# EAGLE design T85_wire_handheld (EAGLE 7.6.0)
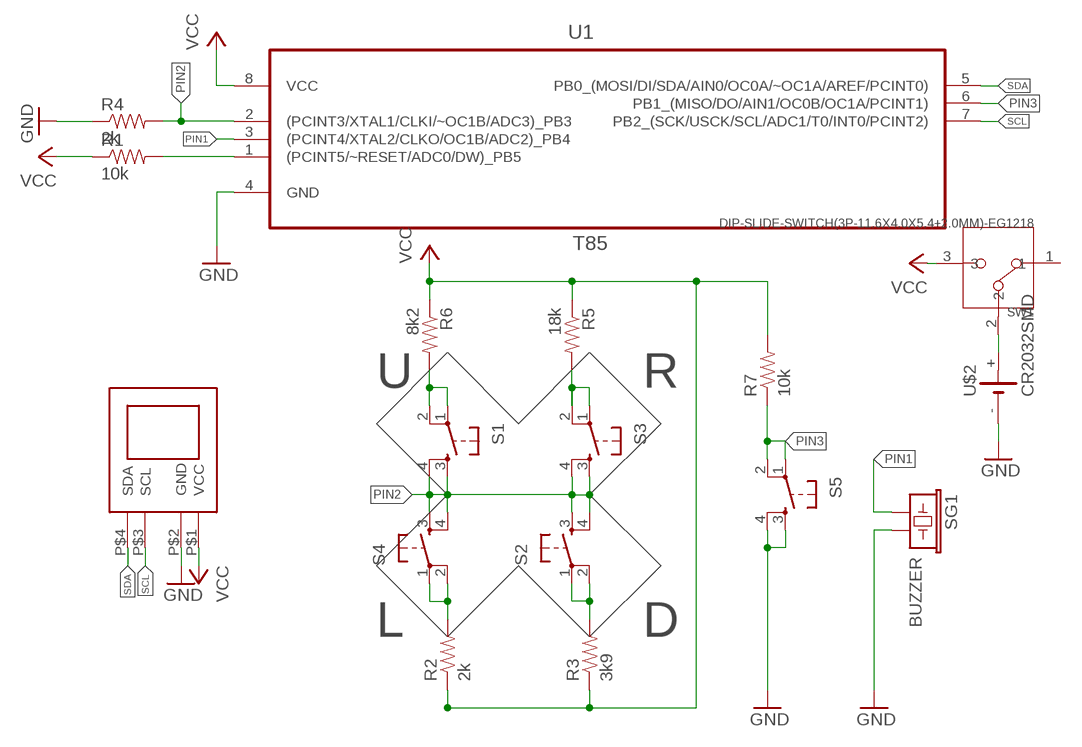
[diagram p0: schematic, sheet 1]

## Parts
R1  10k  RESISTOREZ  [AXIAL-0.3EZ]
R2  2k  RESISTOREZ  [AXIAL-0.3EZ]
R3  3k9  RESISTOREZ  [AXIAL-0.3EZ]
R4  2k  RESISTOREZ  [AXIAL-0.3EZ]
R5  18k  RESISTOREZ  [AXIAL-0.3EZ]
R6  8k2  RESISTOREZ  [AXIAL-0.3EZ]
R7  10k  RESISTOREZ  [AXIAL-0.3EZ]
S1  TAC_SWITCHPTH  [TACTILE-PTH]
S2  TAC_SWITCHPTH  [TACTILE-PTH]
S3  TAC_SWITCHPTH  [TACTILE-PTH]
S4  TAC_SWITCHPTH  [TACTILE-PTH]
S5  TAC_SWITCHPTH  [TACTILE-PTH]
SG1  BUZZER  BUZZERNS  [BUZZER-12MM-NS]
SW1  DIP-SLIDE-SWITCH(3P-11.6X4.0X5.4+2.0MM)-EG1218  [SW3-2.5-11.6X4.0X5.4+2.0MM]
U1  T85  MCU-ATTINY85-20PU(DIP8)1  [DIP254P762X533-8]
U$1  OLED_I2C_VGCD  [OLED_1.3]
U$2  CR2032SMD  [CR2032SMD]

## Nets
GND: R4.P$1 S5.3 S5.4 SG1.- U1.4(GND) U$1.P$2(GND) U$2.-
N$1: R6.P$2 S1.1 S1.2
N$2: R5.P$2 S3.1 S3.2
N$3: SW1.2 U$2.+
N$10: R3.P$2 S2.1 S2.2
N$11: R1.P$2 U1.1((PCINT5/~RESET/ADC0/DW)_PB5)
N$12: R2.P$2 S4.1 S4.2
PIN1: SG1.+ U1.3((PCINT4/XTAL2/CLKO/OC1B/ADC2)_PB4)
PIN2: R4.P$2 S1.3 S1.4 S2.3 S2.4 S3.3 S3.4 S4.3 S4.4 U1.2((PCINT3/XTAL1/CLKI/~OC1B/ADC3)_PB3)
PIN3: R7.P$1 S5.1 S5.2 U1.6(PB1_(MISO/DO/AIN1/OC0B/OC1A/PCINT1))
SCL: U1.7(PB2_(SCK/USCK/SCL/ADC1/T0/INT0/PCINT2)) U$1.P$3(SCL)
SDA: U1.5(PB0_(MOSI/DI/SDA/AIN0/OC0A/~OC1A/AREF/PCINT0)) U$1.P$4(SDA)
VCC: R1.P$1 R2.P$1 R3.P$1 R5.P$1 R6.P$1 R7.P$2 SW1.3 U1.8(VCC) U$1.P$1(VCC)
Unconnected: SW1.1

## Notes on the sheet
- U | R
- L | D

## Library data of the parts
R1-R7 = SparkFun-Passives:RESISTOR: Resistor
S1-S5 = SparkFun-Electromechanical:TAC_SWITCH: Momentary Switch Button commonly used for reset or general input. Spark Fun Electronics SKU : COM-00097 SMT- SWCH-08247
SG1 = SparkFun-Electromechanical:BUZZER: Buzzer 12mm
SW1 = Seeed-OPL-Switch:DIP-SLIDE-SWITCH(3P-11.6X4.0X5.4+2.0MM): 311010006
U1 = Seeed-OPL-ic:MCU-ATTINY85-20PU(DIP8): 310010112; MPN: ATTINY85-20PU; VALUE: ATTINY85-20PU-DIP8
U$1 = oled:OLED_I2C_VGCD
U$2 = battery:CR2032SMD

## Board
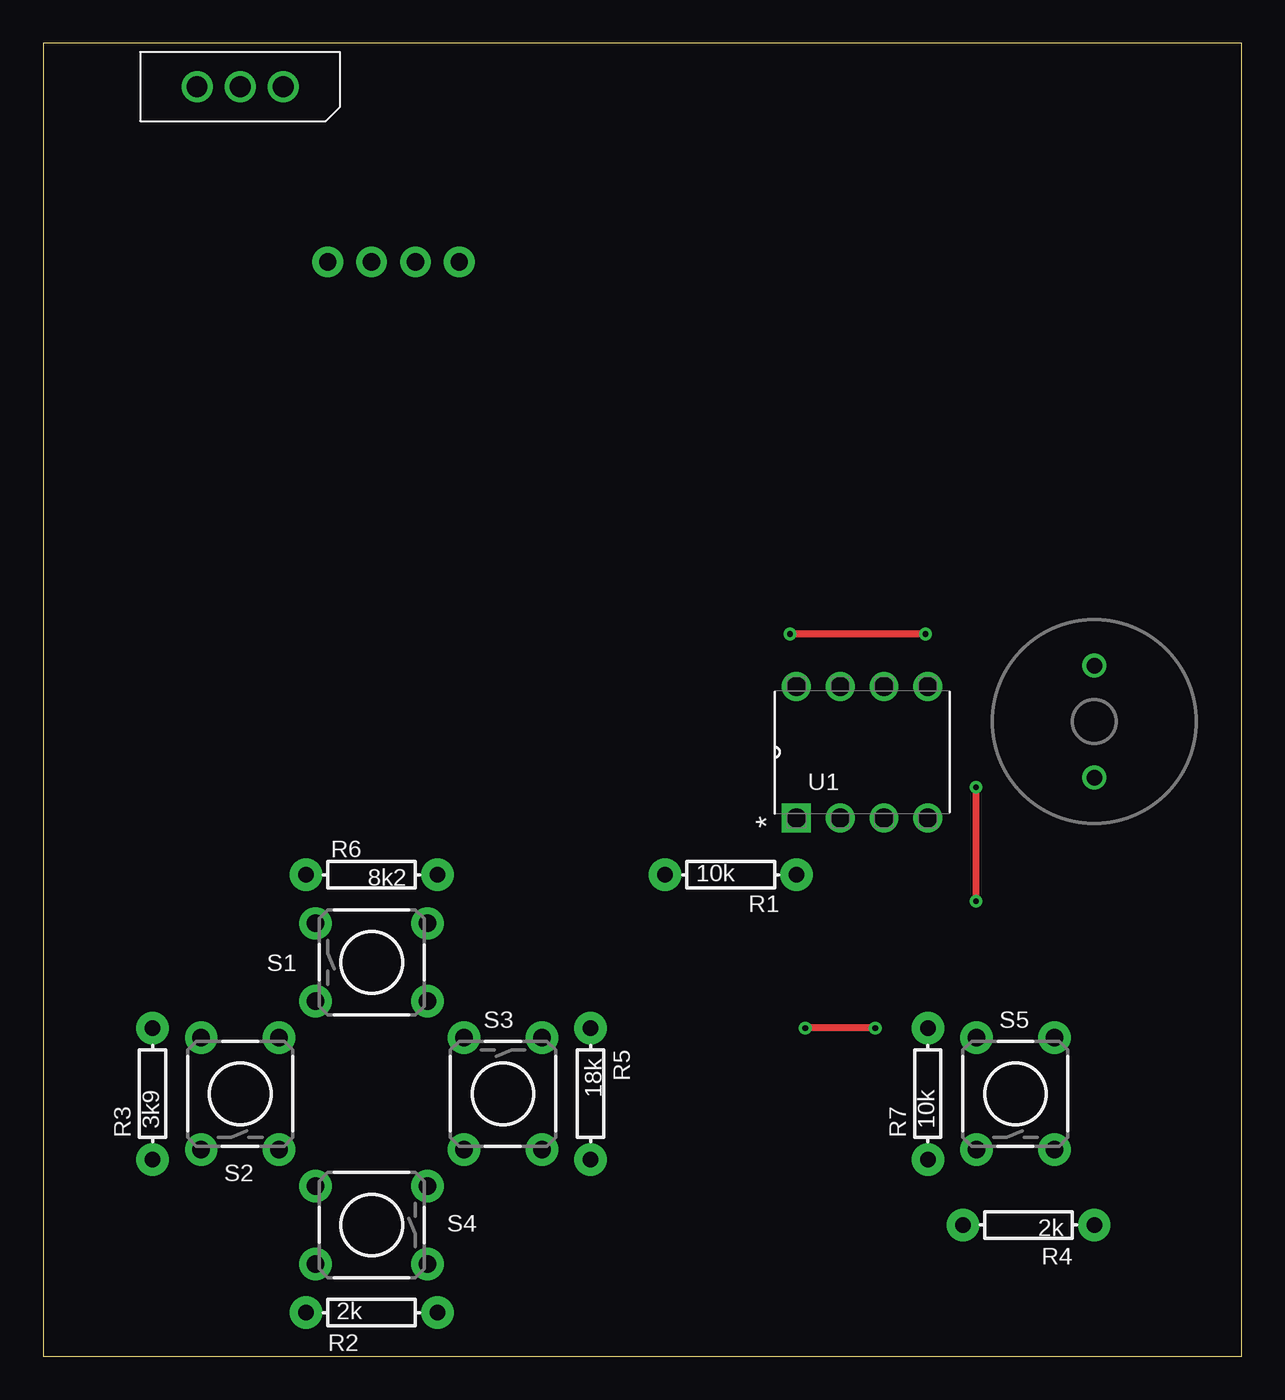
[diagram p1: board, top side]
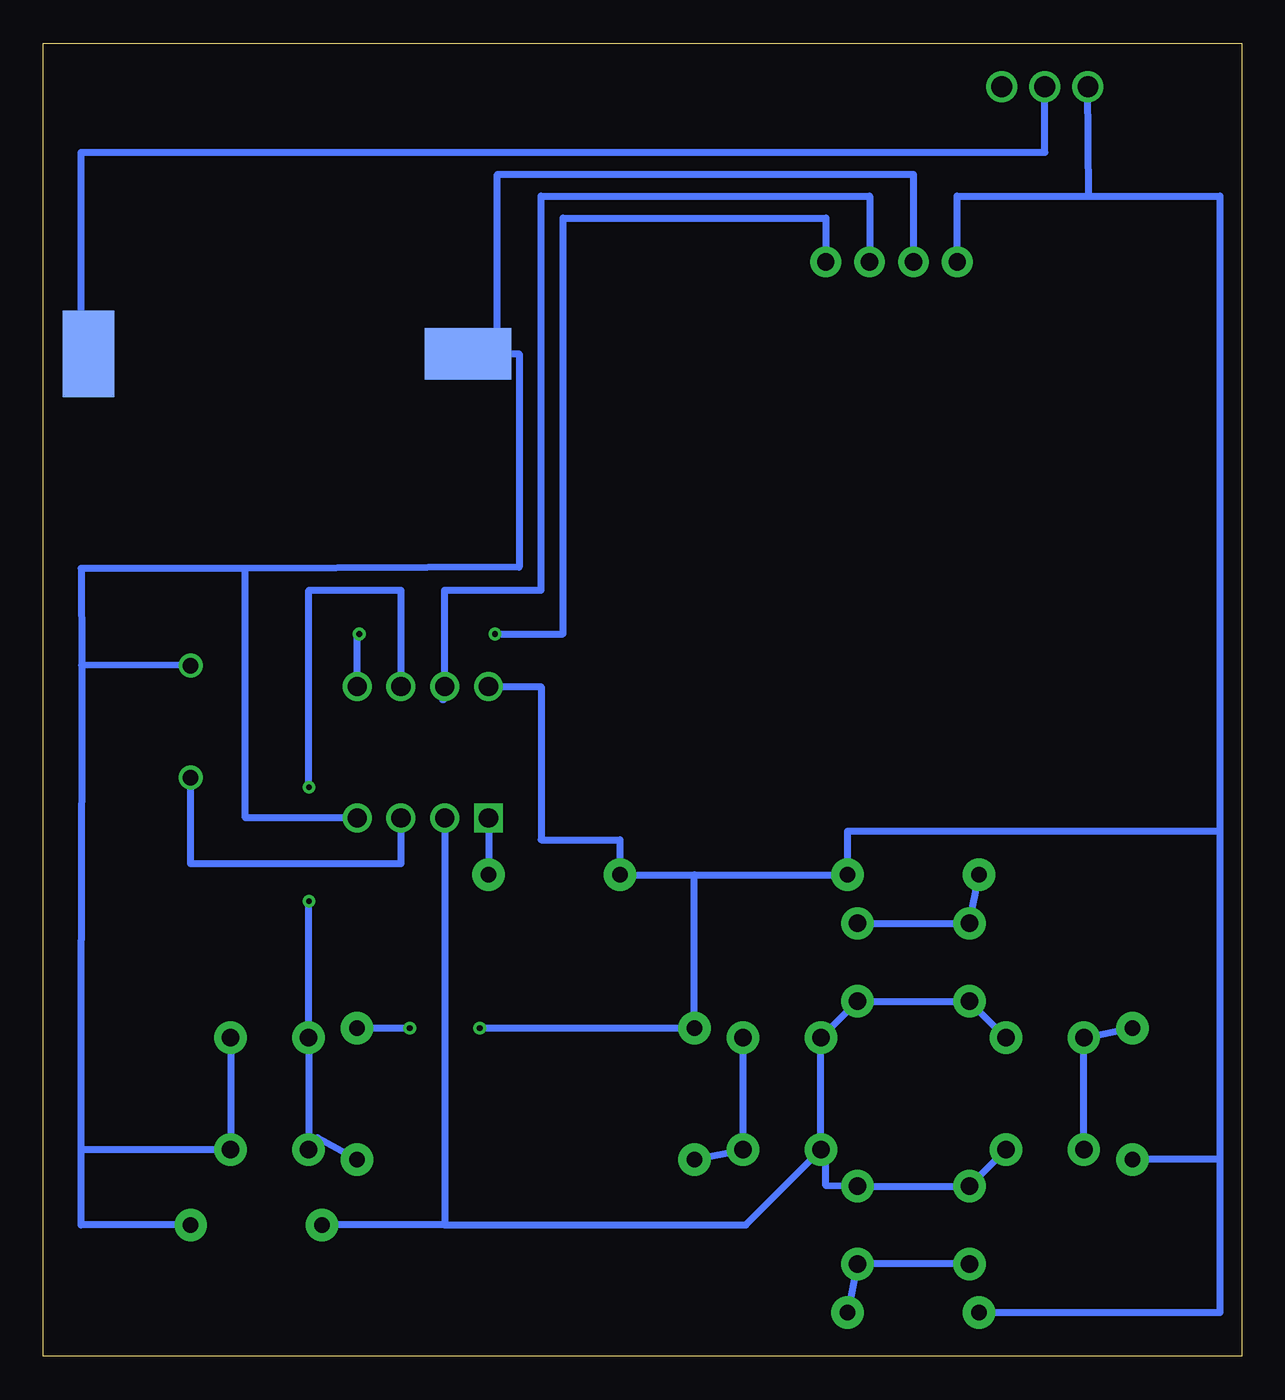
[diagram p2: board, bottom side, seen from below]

Size 69.52 x 76.19 mm. Coordinates in mm from the lower left corner, seen from the top.
Outline: 0,0 69.52,0 69.52,76.19 0,76.19 0,0
Copper layers (1*16): Top 0.035mm / dielectric 1.5mm / Bottom 0.035mm
Design rules "default": minimum track width 10mil, minimum drill 24mil, track to track 8mil, track to pad 8mil, pad to pad 8mil, via to via 8mil, smd to smd 8mil, copper to edge 40mil, drill to drill 8mil, minimum pad ring 10mil, minimum via ring 8mil, stop-mask expansion 4mil, vias tented up to drill 0mil, thermal gap 10mil

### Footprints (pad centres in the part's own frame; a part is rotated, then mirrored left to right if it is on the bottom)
AXIAL-0.3EZ = drill 0.9 pad 1.88: P$1 -3.81,0; P$2 3.81,0
TACTILE-PTH = drill 1.016 pad 1.88: 1 -3.251,2.261; 2 3.251,2.261; 3 -3.251,-2.261; 4 3.251,-2.261
BUZZER-12MM-NS = drill 0.9: + 3.25,0; - -3.25,0
SW3-2.5-11.6X4.0X5.4+2.0MM = drill 1.2: 1 -2.5,0; 2 0,0; 3 2.5,0
DIP254P762X533-8 = drill 1.118 square: 1 -7.62,7.62 | drill 1.118: 2 -7.62,5.08; 3 -7.62,2.54; 4 -7.62,0; 5 0,0; 6 0,2.54; 7 0,5.08; 8 0,7.62
OLED_1.3 = drill 1 pad 1.778: P$1 -3.81,0; P$2 -1.27,0; P$3 1.27,0; P$4 3.81,0
CR2032SMD = smd 5 x 3: + 0,-11 | smd 3 x 5: - 0,11

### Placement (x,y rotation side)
R1  39.88,27.94 0 top
R2  19.05,2.54 0 top
R3  6.35,15.24 90 top
R4  57.15,7.62 180 top
R5  31.75,15.24 270 top
R6  19.05,27.94 180 top
R7  51.31,15.24 90 top
S1  19.05,22.86 0 top
S2  11.43,15.24 90 top
S3  26.67,15.24 270 top
S4  19.05,7.62 180 top
S5  56.39,15.24 90 top
SG1  60.96,36.83 270 top
SW1  11.43,73.66 180 top
U1  51.31,38.86 90 top
U$1  20.32,63.5 0 top
U$2  55.88,58.17 270 bottom

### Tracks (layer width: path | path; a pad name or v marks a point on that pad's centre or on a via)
GND
  Bottom 0.406: S5.4 S5.3 67.31,11.98 | 57.78,45.72 41.91,45.78 41.91,58.17 U$2.- arc90 44.63,57.15 43.43,57.15 arc-90 43.18,57.4 43.18,68.58 19.05,68.58 U$1.P$2 | 57.78,45.72 67.31,45.72 67.29,40.1 | 67.29,40.1 67.31,24.13 67.31,11.98 | SG1.- 67.29,40.1 | 67.31,11.98 67.31,7.62 R4.P$1 | U1.4 57.78,31.24 57.78,45.72
N$1
  Bottom 0.406: S1.2 S1.1 R6.P$2
N$2
  Bottom 0.406: R5.P$2 S3.2 S3.1
N$3
  Bottom 0.406: U$2.+ 67.31,58.17 67.31,69.85 11.43,69.85 SW1.2
N$10
  Bottom 0.406: S2.1 S2.2 R3.P$2
N$11
  Bottom 0.406: U1.1 R1.P$2
N$12
  Bottom 0.406: S4.2 S4.1 R2.P$2
PIN1
  Bottom 0.406: U1.3 48.77,28.57 60.96,28.57 SG1.+
PIN2
  Bottom 0.406: S2.3 S4.4 S4.3 24.13,9.91 24.13,11.99 S3.4 | S3.4 S3.3 S1.4 S1.3 S2.4 | S3.4 28.77,7.62 46.23,7.62 | U1.2 46.23,7.62 | 46.23,7.62 R4.P$2
PIN3  (via drill 0.33)
  Top 0.406: v54.1,26.42 v54.1,33.02
  Bottom 0.406: R7.P$1 53.62,12.7 S5.1 S5.2 54.13,21.84 v54.1,26.42 | v54.1,33.02 54.1,44.45 48.77,44.45 U1.6
SCL
  Bottom 0.406: U1.7 46.35,38.1 arc-90 46.23,38.23 46.23,44.45 40.64,44.45 40.64,67.31 21.59,67.31 U$1.P$3
SDA  (via drill 0.33)
  Top 0.406: v51.18,41.91 v43.31,41.91
  Bottom 0.406: U1.5 51.31,41.66 v51.18,41.91 | v43.31,41.91 39.37,41.91 39.37,66.04 24.13,66.04 U$1.P$4
VCC  (via drill 0.33)
  Top 0.406: v48.26,19.05 v44.2,19.05
  Bottom 0.406: 1.27,11.43 1.27,2.54 R2.P$1 | 1.27,30.48 22.86,30.48 R6.P$1 31.75,27.94 | 1.27,30.48 1.27,11.43 | 1.27,11.43 R3.P$1 | 8.89,67.31 16.51,67.31 U$1.P$1 | 8.89,67.31 SW1.3 | 8.89,67.31 1.27,67.31 1.27,30.48 | U1.8 40.64,38.86 40.64,29.97 36.07,29.97 R1.P$1 31.75,27.94 | R7.P$2 v48.26,19.05 | v44.2,19.05 R5.P$1 31.75,27.94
